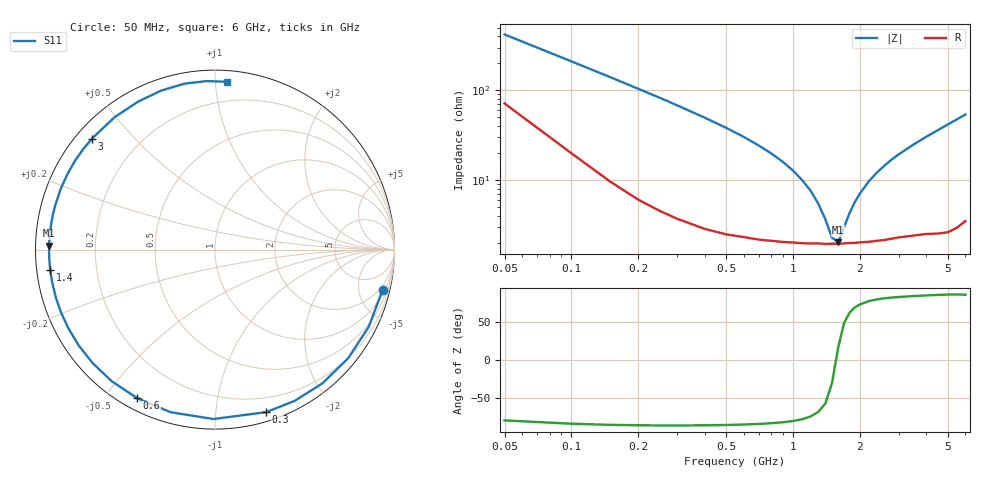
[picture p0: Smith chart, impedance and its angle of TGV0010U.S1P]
! SIEMENS Discrete & RF Semiconductors
! BAT64
! Si Schottky Diode in SOT23
! IF = 0.01 mA
! S-Parameters:  February  1997
# GHz  S  MA  R  50
!  f  S11
! GHz  MAG  ANG
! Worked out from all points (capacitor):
!   34 points, 50 MHz to 6 GHz, reference 50 ohm
!   read as one part to ground: C = 7.56 pF near 50 MHz
!   lowest |Z| = 2.03 ohm at 1.6 GHz (marker M1)
!   series resonance near 1.568 GHz, so ESL is about 1.4 nH
!   S11 on the Smith chart (normalised r, x): 50 MHz: 1.43, -8.27; 300 MHz: 0.07, -1.36; 600 MHz: 0.05, -0.60; 1.4 GHz: 0.04, -0.06; 3 GHz: 0.05, +0.38; 6 GHz: 0.07, +1.07
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0.05  0.9608 -13.4
0.1  0.9584 -26.6
0.15  0.9576 -39.2
0.2  0.9556 -51.2
0.25  0.9526 -62.2
0.3  0.9494 -72.5
0.4  0.944 -90.5
0.5  0.9392 -105.3
0.6  0.9344 -117.7
0.7  0.9321 -128.2
0.8  0.9297 -137.1
0.9  0.9284 -144.8
1  0.9271 -151.6
1.1  0.9266 -157.8
1.2  0.926 -163.2
1.4  0.9255 -172.9
1.6  0.925 178.7
1.8  0.9241 171.3
2  0.9237 164.7
2.4  0.9235 152.9
2.6  0.9237 147.6
3  0.9231 137.9
3.5  0.9257 127.2
4  0.9293 117.4
4.5  0.9353 108.7
5  0.94 100.4
5.5  0.9399 92.8
6  0.9372 85.9
